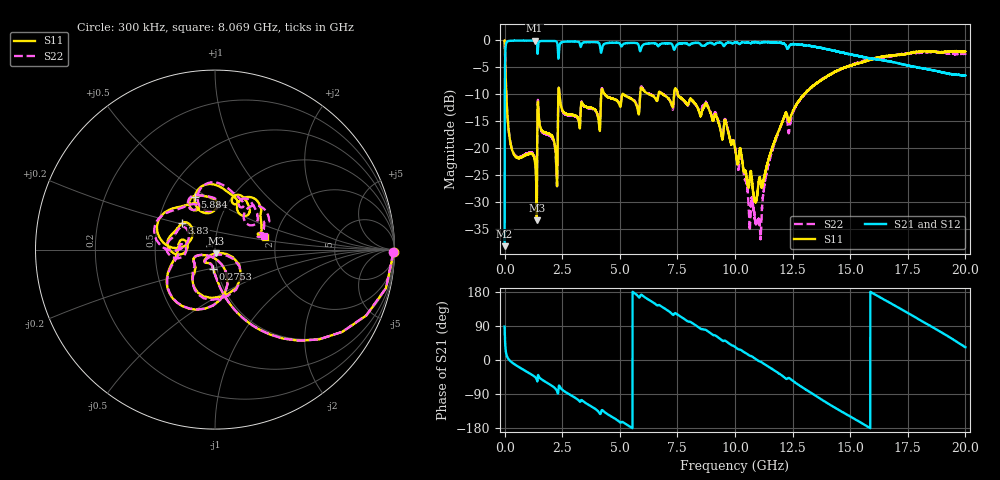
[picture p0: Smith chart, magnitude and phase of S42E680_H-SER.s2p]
!{S42E680}
!Johanson Technology Inc.
!www.johansontechnology.com
!Test Board Conditions:
!Substrate Type  RO4350B
!Substrate Thickness  50 mil
!Substrate Dk  3.66
!TL Type: GCPW
!TL Trace Width  60 mil
!TL Gap  10 mil
!Electrode orientation  Horizontal
!DUT TOPOLOGY	SERIES
!Mounting Pad LxW  14x55 mil
! Created Wed Nov 25 22:24:25 2020
# khz S ma R 50
! 2 Port Network Data from SP1.SP block
! freq  magS11  angS11  magS21  angS21  magS12  angS12  magS22  angS22
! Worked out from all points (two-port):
!   20001 points, 300 kHz to 20 GHz, reference 50 ohm
!   highest |S21| = -0.04 dB at 1.3 GHz (marker M1); lowest = -38.1 dB at 300 kHz (marker M2)
!   |S21| within 3 dB of the highest: 24.1 MHz to 2.327 GHz (2.303 GHz wide, 196 % of centre); 2.347 GHz to 15.51 GHz (13.17 GHz wide, 147 % of centre)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
!   lowest |S11| = -33.3 dB at 1.396 GHz (marker M3), VSWR 1.04, Z = 50.5 - j2.11 ohm
!   |S11| at or under -10 dB: 73.34 MHz to 2.331 GHz (2.258 GHz wide, 188 % of centre); 2.384 GHz to 4.194 GHz (1.81 GHz wide, 55 % of centre); 7.505 GHz to 13 GHz (5.49 GHz wide, 53.6 % of centre)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
!   |S22| runs from -36.9 to 0.0 dB; largest |S21 - S12| = 0.02
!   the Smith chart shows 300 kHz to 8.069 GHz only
!   S11 on the Smith chart (normalised r, x): 300 kHz: open; 275.3 MHz: 0.96, -0.20; 3.83 GHz: 0.66, +0.21; 5.884 GHz: 0.68, +0.44; 8.069 GHz: 1.75, +0.27
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300  0.9957 -0.8  0.01241 88.2  0.01249 89.1  0.9937 -0.8
105300  0.2296 -80.9  0.972 9.4  0.9715 9.3  0.2307 -80.9
275300  0.1059 -95.9  0.991 -4.2  0.9912 -4.2  0.1073 -95.9
1300300  0.07965 -135.6  0.9956 -43.8  0.9945 -43.8  0.0826 -132.2
1396300  0.0216 -75.0  0.9745 -51.4  0.9736 -51.4  0.03036 -74.0
1520300  0.167 -132.7  0.9804 -47.0  0.9798 -46.9  0.1634 -137.1
2205300  0.09836 -160.9  0.9847 -75.5  0.9857 -75.4  0.09355 -160.7
2415300  0.2724 -158.0  0.9372 -72.7  0.9362 -72.7  0.2685 -157.5
3334300  0.2666 173.2  0.9043 -105.5  0.9043 -105.6  0.2709 178.8
3830300  0.2345 141.4  0.9643 -125.0  0.9659 -125.0  0.231 149.0
4912300  0.2715 110.2  0.9514 -159.5  0.9501 -159.5  0.2731 113.1
5884300  0.3151 111.0  0.7931 168.7  0.7928 168.7  0.3272 106.7
6667300  0.3111 71.0  0.8821 144.7  0.8793 144.6  0.3121 62.7
8069300  0.2885 14.2  0.9227 100.5  0.9186 100.7  0.2851 14.9
1.00003e7  0.09992 -41.1  0.9583 34.5  0.9589 34.5  0.1014 -61.1
1.10483e7  0.05229 34.4  0.9499 -3.2  0.9484 -3.1  0.02145 102.3
1.20463e7  0.1734 47.8  0.9431 -41.3  0.9436 -41.3  0.173 42.4
1.33343e7  0.37 7.1  0.8832 -88.0  0.8842 -87.9  0.3697 -3.7
1.49933e7  0.5827 -56.6  0.7444 -148.9  0.7416 -149.2  0.5844 -61.6
1.66673e7  0.7166 -112.3  0.6429 153.0  0.6281 153.0  0.7114 -120.8
1.84783e7  0.786 -175.5  0.5361 89.8  0.5348 90.4  0.7815 -178.6
2e7  0.7878 137.4  0.4712 33.7  0.4747 34.4  0.7494 125.0
